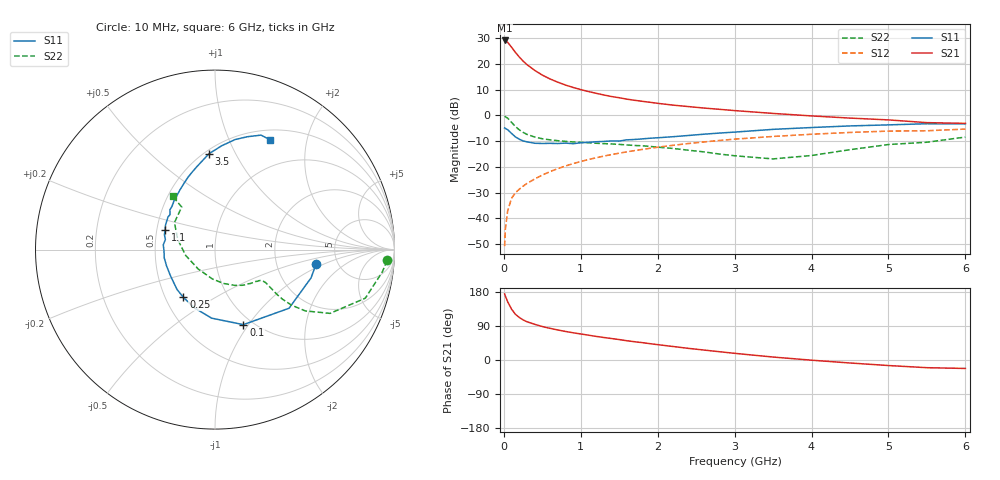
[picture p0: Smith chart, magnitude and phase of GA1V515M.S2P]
! Infineon Technologies  Discrete & RF Semiconductors
! BF775
! Si NPN RF Bipolar Junction Transistor in SOT23
! VCE = 1.5 V  IC = 15 mA
! Common Emitter S-Parameters:  May  1996
# GHz  S  MA  R  50
!  f  S11  S21  S12  S22
! GHz  MAG  ANG  MAG  ANG  MAG  ANG  MAG  ANG
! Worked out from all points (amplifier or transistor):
!   36 points, 10 MHz to 6 GHz, reference 50 ohm
!   highest |S21| = 29.1 dB at 10 MHz (marker M1)
!   |S21| within 3 dB of that: start of sweep to 109.9 MHz
!   unconditionally stable (mu >= 1): 385 MHz to 4.316 GHz; 5.146 GHz to end of sweep
!   at 250 MHz: K = 0.85, MSG = 24.3 dB, |S12| = -27.5 dB
!   at 1.4 GHz: K = 1.15, MAG = 8.9 dB, |S12| = -15.2 dB
!   at 6 GHz: K = 1.01, MAG = 0.5 dB, |S12| = -5.3 dB
!   S11 on the Smith chart (normalised r, x): 10 MHz: 3.42, -0.82; 100 MHz: 0.91, -0.95; 250 MHz: 0.62, -0.37; 1.1 GHz: 0.55, +0.14; 3.5 GHz: 0.53, +0.79; 6 GHz: 0.62, +1.44
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0.01  0.5689 -8.2  28.37 174.4  0.0029 87.1  0.9609 -3.6
0.02  0.5579 -16.4  28.11 168.5  0.0062 83.5  0.9405 -7.6
0.05  0.5262 -38.4  26.03 153.5  0.0141 74.2  0.8802 -17.9
0.1  0.4469 -69.3  21.03 134.3  0.0245 66.8  0.733 -29.0
0.15  0.3824 -92.8  16.67 120.8  0.0315 62.5  0.6078 -34.2
0.2  0.3446 -109.3  13.6 112.3  0.0368 61.4  0.5252 -36.0
0.25  0.3191 -123.5  11.29 105.9  0.0423 62.5  0.4678 -36.3
0.3  0.3065 -133.8  9.67 101.0  0.0477 63.2  0.4278 -35.9
0.4  0.2876 -149.9  7.479 94.2  0.0582 64.7  0.3801 -34.6
0.5  0.2848 -161.1  6.041 88.3  0.0695 65.9  0.3518 -33.6
0.6  0.2866 -171.0  5.091 83.6  0.0809 66.5  0.3346 -33.1
0.7  0.284 -178.4  4.407 79.3  0.0924 66.7  0.3227 -33.2
0.8  0.2894 174.8  3.88 75.4  0.104 65.9  0.3128 -33.6
0.9  0.2822 168.5  3.479 71.9  0.1158 65.6  0.3052 -34.3
1.1  0.2994 158.1  2.898 65.5  0.1391 64.3  0.2942 -36.9
1.3  0.3121 149.6  2.481 59.4  0.1623 62.4  0.283 -39.8
1.6  0.335 138.6  2.06 50.8  0.196 59.2  0.2665 -45.6
2.2  0.3855 120.5  1.579 35.6  0.2625 51.8  0.2279 -61.0
3.5  0.5351 93.6  1.09 7.8  0.3896 33.7  0.1429 -131.1
4.5  0.6236 79.6  0.885 -7.9  0.466 19.8  0.2158 164.6
5.5  0.6874 68.1  0.722 -20.3  0.5026 5.6  0.3011 128.0
6  0.6844 63.2  0.699 -22.3  0.5415 1.5  0.3794 128.5
